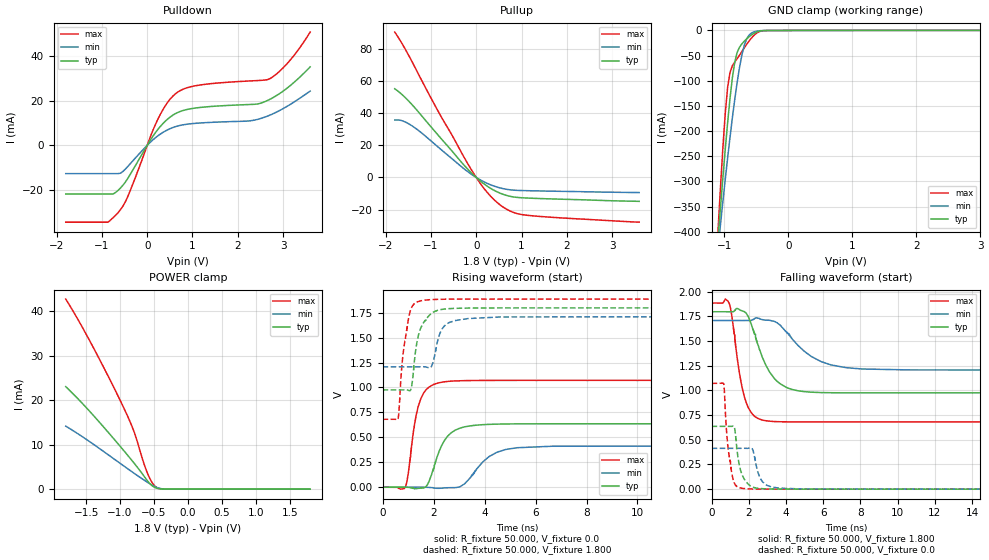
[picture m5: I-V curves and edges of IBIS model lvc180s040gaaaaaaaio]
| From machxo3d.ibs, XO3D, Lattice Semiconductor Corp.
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|   Model lvc180s040gaaaaaaaio
[Model] lvc180s040gaaaaaaaio
Model_type I/O
Polarity   Non-Inverting
Enable   Active-Low
Vinl =  0.630V
Vinh =  1.170V
Vmeas =  0.900V
Cref =  0.0F
Rref =  1.000M
Vref =  0.0V
C_comp   4.200pF   3.800pF   7.500pF
[Temperature Range]   25.000   0.105k   -40.000
[Voltage Range]   1.800V   1.710V   1.890V
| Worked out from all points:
|   slope of the pulldown table from 0 to 0.27 V, typ, clamps not added: 34 ohm
|   slope of the pullup table from 0 to 0.27 V, typ, clamps not added: 45.6 ohm
|   GND clamp passes 1 mA (typ) near -0.44 V on its own axis
|   POWER clamp passes 1 mA (typ) near -0.55 V on its own axis
|   rising waveform, R_fixture 50.000, V_fixture 0.0: 20-80 % time 620ps typ, 954ps min, 412ps max; typ from 0 V to 0.636 V
|   rising waveform, R_fixture 50.000, V_fixture 1.800: 20-80 % time 366ps typ, 368ps min, 307ps max; typ from 0.976 V to 1.8 V
|   falling waveform, R_fixture 50.000, V_fixture 1.800: 20-80 % time 1.1ns typ, 1.8ns min, 619ps max; typ from 1.8 V to 0.976 V
|   falling waveform, R_fixture 50.000, V_fixture 0.0: 20-80 % time 378ps typ, 404ps min, 321ps max; typ from 0.636 V to 0 V
[Pulldown]
|Voltage   I(typ)   I(min)   I(max)
-1.8V     -21.78mA   -12.65mA   -34.34mA
-865mV    -21.78mA   -12.65mA   -34.34mA
-645mV    -20.15mA   -12.65mA   -30.11mA
-425mV    -14.65mA   -9.378mA   -22.7mA
235mV     7.083mA    4.214mA    11.64mA
455mV     11.78mA    6.962mA    19.3mA
620mV     14.1mA     8.304mA    22.95mA
1.115V    16.77mA    9.887mA    26.76mA
2.27V     18.22mA    10.93mA    28.74mA
2.71V     20.53mA    13.47mA    29.76mA
3.15V     26.5mA     18.13mA    37.84mA
3.6V      35.01mA    24.22mA    50.56mA
[Pullup]
|Voltage   I(typ)   I(min)   I(max)
-1.8V     55.05mA    35.68mA    90.21mA
-1.625V   51.08mA    35.09mA    82.4mA
-1.35V    43.03mA    30.71mA    68.13mA
-800mV    24.9mA     17.87mA    38.97mA
-140mV    3.787mA    2.633mA    6.305mA
25mV      -631.9uA   -432.1uA   -1.07mA
190mV     -4.372mA   -2.969mA   -7.464mA
355mV     -7.378mA   -4.969mA   -12.72mA
520mV     -9.667mA   -6.446mA   -16.87mA
795mV     -11.95mA   -7.796mA   -21.4mA
1.07V     -12.7mA    -8.16mA    -23.29mA
3.6V      -14.81mA   -9.369mA   -27.75mA
[GND_clamp]
|Voltage   I(typ)   I(min)   I(max)
-1.8V     -1.677A    -1.372A    -2.207A
-1.097V   -411.7mA   -430.5mA   -393mA
-1.06V    -351mA     -384.7mA   -309.9mA
-986mV    -235.9mA   -295.9mA   -164.8mA
-949mV    -183mA     -253.4mA   -113.1mA
-912mV    -135mA     -212.5mA   -83.39mA
-838mV    -63.2mA    -137.2mA   -62.73mA
-801mV    -43.97mA   -103.8mA   -56.32mA
-690mV    -21.54mA   -30.09mA   -34.79mA
-579mV    -9.102mA   -5.388mA   -15.4mA
-357mV    -191.3uA   -96.81uA   -298.1uA
3.6V      109.7uA    43.11uA    257.2uA
[POWER_clamp]
|Voltage   I(typ)   I(min)   I(max)
-1.8V     23.01mA    14.15mA    42.67mA
-1.641V   20.61mA    12.64mA    38.63mA
-1.456V   17.62mA    10.75mA    33.57mA
-1.012V   9.864mA    5.936mA    20.36mA
-864mV    7.162mA    4.325mA    15.53mA
-790mV    5.771mA    3.533mA    12.74mA
-679mV    3.583mA    2.37mA     7.204mA
-605mV    2.041mA    1.626mA    3.889mA
-531mV    791.7uA    936.7uA    1.526mA
-457mV    198.5uA    375.7uA    334.5uA
-272mV    2.958uA    5.534uA    1.322uA
1.8V      0A         0A         0A
[Ramp]
| variable   typ   min   max
dV/dt_r   0.382/0.630n   0.248/0.933n   0.643/0.410n
dV/dt_f   0.493/1.096n   0.301/1.778n   0.723/0.620n
R_load = 50.000
[Rising Waveform]
R_fixture= 50.000
V_fixture= 0.0
V_fixture_min= 0.0
V_fixture_max= 0.0
|time   V(typ)   V(min)   V(max)
0s        4.637nV    47.96nV    2.735nV
899ps     113uV      2.085uV    2.593mV
1.257ns   -15.53mV   116.9uV    634.6mV
1.403ns   -10.99mV   295uV      813mV
1.758ns   24.88mV    -921.6uV   989.3mV
2.221ns   361.5mV    -10.81mV   1.047V
3.026ns   591.5mV    3.183mV    1.067V
4.181ns   630.3mV    307.7mV    1.071V
5.273ns   635.3mV    396mV      1.071V
20ns      636.4mV    413.8mV    1.071V
[Rising Waveform]
R_fixture= 50.000
V_fixture= 1.800
V_fixture_min= 1.710
V_fixture_max= 1.890
|time   V(typ)   V(min)   V(max)
0s        975.6mV    1.207V     681.2mV
608ps     975.6mV    1.207V     685.2mV
807ps     975.6mV    1.207V     1.342V
1.024ns   970.1mV    1.207V     1.698V
1.139ns   1.009V     1.207V     1.801V
1.484ns   1.587V     1.207V     1.867V
1.931ns   1.744V     1.218V     1.88V
2.415ns   1.786V     1.614V     1.884V
3.352ns   1.796V     1.691V     1.886V
20ns      1.798V     1.709V     1.886V
[Falling Waveform]
R_fixture= 50.000
V_fixture= 1.800
V_fixture_min= 1.710
V_fixture_max= 1.890
|time   V(typ)   V(min)   V(max)
0s        1.798V     1.709V     1.886V
961ps     1.797V     1.709V     1.877V
1.461ns   1.824V     1.709V     1.219V
1.758ns   1.799V     1.709V     939mV
2.121ns   1.679V     1.709V     777.6mV
2.722ns   1.339V     1.718V     700.5mV
4.047ns   1.028V     1.585V     682.2mV
5.358ns   982.6mV    1.344V     681.2mV
7.222ns   976mV      1.231V     681.2mV
20ns      975.6mV    1.207V     681.1mV
[Falling Waveform]
R_fixture= 50.000
V_fixture= 0.0
V_fixture_min= 0.0
V_fixture_max= 0.0
|time   V(typ)   V(min)   V(max)
0s        636.4mV    413.8mV    1.071V
653ps     636.4mV    413.8mV    1.066V
825ps     636.4mV    413.8mV    536.3mV
1.055ns   636.5mV    413.8mV    198mV
1.243ns   612mV      413.8mV    54.24mV
1.548ns   197.2mV    413.7mV    12.26mV
2.155ns   25.51mV    416.1mV    1.992mV
2.65ns    6.162mV    98.95mV    442uV
3.616ns   906.8uV    10.62mV    74.41uV
20ns      2.005nV    93.37nV    12.24nV
